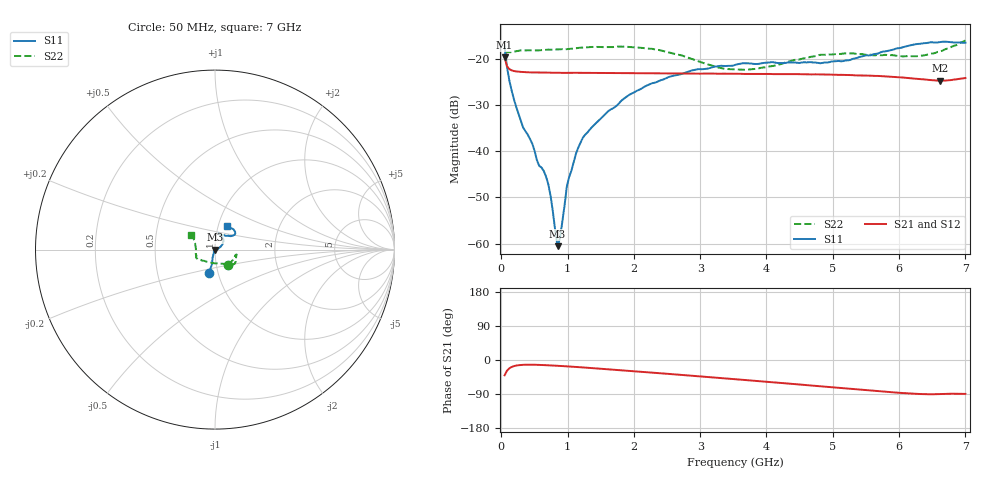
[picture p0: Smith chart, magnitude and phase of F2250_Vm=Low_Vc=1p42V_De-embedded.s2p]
! Integrated Device Technology
! Corporate Headquarters
! 6024 Silver Creek Valley Road
! San Jose, CA 95138  USA
! Phone:  1-408-284-8200
! Toll Free:  1-800-223-1366
! Webpage:  http://www.idt.com/
! Timing and RF Division
! 515 Groton Road, Suite 102
! Westford, MA 01886-6024
! Device:  F2250
! Description: Voltage Variable RF Attenuator
! Frequency:  50.0 -  6000.00 MHz
! Package:  3x3 mm Thin QFN Plastic Package: 16 pin
! Ports:  2 RF, 3 DC
!  Pin  1  = GND
!  Pin  2  = NC
!  Pin  3  = RF1  = Port 1
!  Pin  4  = NC
!  Pin  5  = GND
!  Pin  6  = GND
!  Pin  7  = GND
!  Pin  8  = GND
!  Pin  9  = NC
!  Pin 10  = RF2  = Port 2
!  Pin 11  = NC
!  Pin 12  = GND
!  Pin 13  = GND
!  Pin 14  = VCNTRL
!  Pin 15  = VDD
!  Pin 16  = VMODE
! Vcntrl:  1.420 Volts
! Vmode:  +0.000 Volts
! Vdd:  +3.30  Volts
! Current:  1.191 mA
! Data:  The device was measured on a the F2250 evaluation board which has
!  individual transmission lines to the RF pins.  Data was collected
!  using a calibrated network analyzer.  The evaluation board was
!  de-embedded using a TRL calibration technique.
!  The reference plane is the edge of the package pin.
! Misc:  SN 10
!  Action Tracker AT0258
! Date Measured:  2014-11-26
! Date:  2015-10-15  MJV
! Note:
!  Integrated Device Technology supplies this data as a sample of measured
!  data at the package pin for this product.  Your particular data for this
!  product may vary.
!  Data was taken at 25 degrees C.
!  Integrated Device Technology reserves the right to change this data at anytime.
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# GHz S dB R 50
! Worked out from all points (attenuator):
!   201 points, 50 MHz to 7 GHz, reference 50 ohm
!   highest |S21| = -19.74 dB at 50 MHz (marker M1); lowest = -24.8 dB at 6.618 GHz (marker M2)
!   lowest |S11| = -60.6 dB at 849.2 MHz (marker M3), VSWR 1.00, Z = 50 - j0.0937 ohm
!   |S11| at or under -10 dB: start of sweep to end of sweep
!   |S22| runs from -22.4 to -16.1 dB; largest |S21 - S12| = 0.00024
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0.05  -17.36 -104.8  -19.74 -40.3  -19.73 -40.3  -18.94 -49.0
0.1195  -24.57 -104.0  -22.24 -22.2  -22.23 -22.1  -18.60 -18.7
0.22375  -30.37 -108.1  -22.75 -14.7  -22.75 -14.7  -18.40 -13.8
0.328  -34.85 -112.4  -22.87 -12.7  -22.87 -12.7  -18.20 -12.9
0.467  -38.38 -120.2  -22.97 -12.4  -22.96 -12.4  -18.21 -13.8
0.5365  -41.93 -119.3  -23.00 -12.7  -22.98 -12.7  -18.20 -15.4
0.64075  -44.29 -116.8  -23.01 -13.4  -23.00 -13.4  -18.12 -17.3
0.71025  -47.23 -114.5  -23.02 -14.0  -23.03 -13.9  -18.05 -18.9
0.745  -49.82 -117.1  -23.02 -14.3  -23.03 -14.3  -18.06 -19.6
0.84925  -60.56 -90.2  -23.05 -15.3  -23.04 -15.3  -17.99 -22.0
0.884  -58.91 -32.5  -23.05 -15.6  -23.06 -15.6  -17.96 -22.8
0.98825  -47.70 -18.6  -23.06 -16.7  -23.07 -16.7  -17.94 -24.6
1.12725  -40.50 5.7  -23.06 -18.3  -23.05 -18.3  -17.75 -26.8
1.2315  -37.07 11.7  -23.08 -19.6  -23.07 -19.6  -17.58 -28.8
1.857  -28.57 28.6  -23.13 -27.7  -23.12 -27.7  -17.40 -36.3
2.37825  -24.82 39.4  -23.17 -34.7  -23.18 -34.7  -18.13 -42.5
2.93425  -22.35 54.6  -23.23 -42.3  -23.21 -42.4  -20.36 -56.1
3.525  -21.35 68.8  -23.26 -50.7  -23.26 -50.7  -22.33 -91.9
4.7065  -20.83 70.5  -23.39 -67.8  -23.39 -67.8  -19.53 -148.7
5.85325  -18.21 38.5  -23.88 -84.6  -23.88 -84.6  -19.26 -167.8
6.61775  -16.41 45.2  -24.75 -89.8  -24.75 -89.9  -18.42 159.4
7  -16.54 62.7  -24.18 -89.4  -24.17 -89.5  -16.06 149.4
